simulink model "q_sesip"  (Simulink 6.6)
settings: Solver=FixedStepDiscrete  StartTime=0.0  StopTime=inf  FixedStep=0.002  RelTol=1e-3
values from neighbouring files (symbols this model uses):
  ALPHA_LIM_ENABLE = 1    [setup_srv02_exp08_sip.m]
  ALPHA_MAX = 45    [setup_srv02_exp08_sip.m]
  ALPHA_MIN = - ALPHA_MAX    (= -45)    [setup_srv02_exp08_sip.m]
  CATCH_ALPHA_DOT_LIM = VMAX_AMP/k(4)    [setup_srv02_exp08_sip.m]
  CATCH_ALPHA_UP_LIM = 1.5 * pi / 180    (= 0.0261799387799)    [setup_srv02_exp08_sip.m]
  Er = 0.8    [calculate_qr.m]
  eta_g = 0.90    (= 0.9)    [config_srv02.m]
  eta_m = 0.69    [config_srv02.m]
  g = 9.81    [config_sp.m]    (also in setup_srv02_exp08_sip.m)
  k = zeros(1,4)    [setup_srv02_exp08_sip.m]
  K_AMP = 1    [setup_srv02_exp08_sip.m]
  K_ENC = 0    [config_srv02.m]
  Kg = 0    [config_srv02.m]
  km = 0.804 / 1000 * K_RDPS2RPM    [config_srv02.m]
  kt = 1.088 * K_OZ2N * K_IN2M    [config_srv02.m]
  lp = (2 + 7/16) * K_IN2M    [config_sp.m]
  n = u_max / g    [setup_srv02_exp08_sip.m]
  Rm = 2.6    [config_srv02.m]
  THETA_LIM_ENABLE = 1    [setup_srv02_exp08_sip.m]
  THETA_MAX = 60    [setup_srv02_exp08_sip.m]
  THETA_MIN = - THETA_MAX    (= -60)    [setup_srv02_exp08_sip.m]
  VMAX_AMP = 0    [config_srv02.m]
  VMAX_DAC = 10    [setup_srv02_exp08_sip.m]
  wcf_2 = 2 * pi * 8.5    (= 53.407075111)    [setup_srv02_exp08_sip.m]
undefined symbols (not defined in the file or in its folder): HIL, Jp_cm, l_arm, m_arm, mp, qc_get_step_size
libraries: quarc_library x12, simulink_extras x6, simulink x2

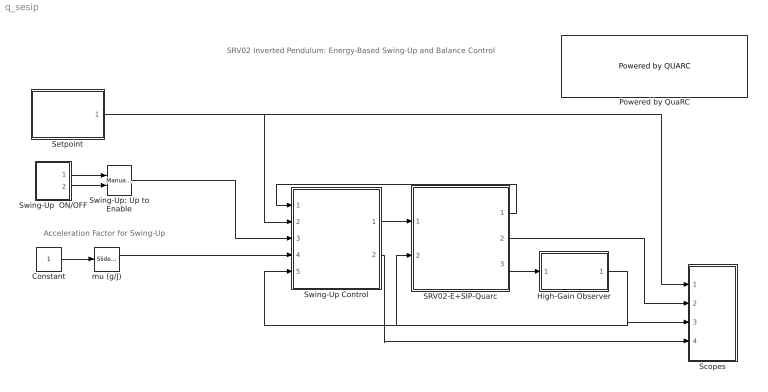
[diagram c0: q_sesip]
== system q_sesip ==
  note: SRV02 Inverted Pendulum: Energy-Based Swing-Up and Balance Control
  note: Acceleration Factor for Swing-Up
  Constant : Constant
  High-Gain Observer : Subsystem
  Powered by QuaRC : quarc_library/Logos/Powered by QUARC  SystemSampleTime=-1
  SRV02-E+SIP-Quarc : Subsystem
  Scopes : Subsystem
  Setpoint : Subsystem
  Swing-Up  ON/OFF : Subsystem
  Swing-Up Control : Subsystem
  Swing-Up: Up to Enable : simulink/Signal Routing/Manual Switch  SystemSampleTime=-1  sw=1  action=0  varsize=off
  mu (g/J) : simulink/Math Operations/Slider Gain  SystemSampleTime=-1  low=0  gain=0.23544  high=1
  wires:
  Swing-Up Control/1(tau (N.m)) -> SRV02-E+SIP-Quarc/1(tau (N.m))
  SRV02-E+SIP-Quarc/3(Y) -> High-Gain Observer/1(Y)
  Setpoint/1(Xd) -> Scopes/1(X_d), Swing-Up Control/2(Xd)
  SRV02-E+SIP-Quarc/1(a_f (rad)) -> Swing-Up Control/1(a_f (rad))
  Swing-Up  ON/OFF/1(on) -> Swing-Up: Up to Enable/1
  Swing-Up  ON/OFF/2(off) -> Swing-Up: Up to Enable/2
  Swing-Up: Up to Enable/1 -> Swing-Up Control/3(swing on/off)
  Swing-Up Control/2(E (J)) -> Scopes/4(E)
  SRV02-E+SIP-Quarc/2(Vm (V)) -> Scopes/2(Vm)
  High-Gain Observer/1(Xe) -> Swing-Up Control/5(X), SRV02-E+SIP-Quarc/2(X), Scopes/3(X)
  Constant/1 -> mu (g/J)/1
  mu (g/J)/1 -> Swing-Up Control/4(mu (g/J))

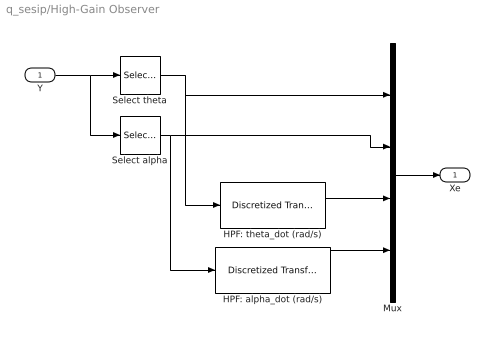
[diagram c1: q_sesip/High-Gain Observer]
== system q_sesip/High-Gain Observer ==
  Y : Inport
  HPF: alpha_dot (rad/s) : quarc_library/Discrete/Discretized Transfer Function  SystemSampleTime=-1  num=[wcf_2 0]  den=[1 wcf_2]  method=tustin  Ts=qc_get_step_size
  HPF: theta_dot (rad/s) : quarc_library/Discrete/Discretized Transfer Function  SystemSampleTime=-1  num=[100 0]  den=[1 100]  method=tustin  Ts=qc_get_step_size
  Mux : Mux
  Select alpha : Selector  IndexOptions=Index vector (dialog)  Indices=2  OutputSizes=1  InputPortWidth=2
  Select theta : Selector  IndexOptions=Index vector (dialog)  Indices=1  OutputSizes=1  InputPortWidth=2
  Xe : Outport
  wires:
  Select alpha/1 -> Mux/2, HPF: alpha_dot (rad/s)/1
  Mux/1 -> Xe/1
  Y/1 -> Select alpha/1, Select theta/1
  HPF: theta_dot (rad/s)/1 -> Mux/3
  Select theta/1 -> Mux/1, HPF: theta_dot (rad/s)/1
  HPF: alpha_dot (rad/s)/1 -> Mux/4

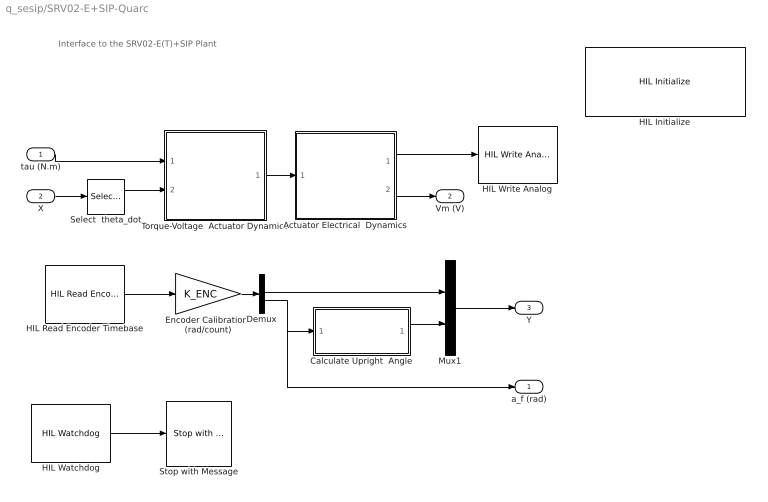
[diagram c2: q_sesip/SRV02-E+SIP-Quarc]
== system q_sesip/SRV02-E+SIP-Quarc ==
  note: Interface to the SRV02-E(T)+SIP Plant
  tau (N.m) : Inport
  X : Inport  Port=2
  Actuator Electrical  Dynamics : Subsystem
  Calculate Upright  Angle : Subsystem
  Demux : Demux  Outputs=2
  Encoder Calibration  (rad/count) : Gain  Gain=K_ENC
  HIL Initialize : quarc_library/Data Acquisition/Generic/Configuration/HIL Initialize  object_name=HIL-1  board_type=q8  board_number=0  exclusive=off  active=on  hardware_clocks=0:1  clock_modes=[0 0]  set_clock_params_at_start=on  set_clock_params_at_switch_in=off  analog_input_channels=0:7  analog_input_maximums=10  analog_input_minimums=-10  set_analog_input_params_at_start=on  set_analog_input_params_at_switch_in=off  analog_output_channels=0:7  analog_output_maximums=10  analog_output_minimums=-10  initial_analog_outputs=0  final_analog_outputs=0  watchdog_analog_outputs=0  set_analog_output_params_at_start=on  set_analog_output_params_at_switch_in=off  set_analog_outputs_at_start=on  set_analog_outputs_at_switch_in=off  set_analog_outputs_at_terminate=on  set_analog_outputs_at_switch_out=off  set_analog_outputs_on_watchdog=on  digital_input_channels=[]  digital_output_channels=[]  digital_output_configuration=[]  initial_digital_outputs=1  final_digital_outputs=1  watchdog_digital_outputs=0  set_digital_output_params_at_start=off  set_digital_output_params_at_switch_in=off  set_digital_outputs_at_start=on  set_digital_outputs_at_switch_in=off  set_digital_outputs_at_terminate=on  set_digital_outputs_at_switch_out=off  set_digital_outputs_on_watchdog=off  encoder_channels=0:7  quadrature=4  encoder_filter_frequency=(1/120e-9)/1  initial_encoder_counts=0  set_encoder_params_at_start=on  set_encoder_params_at_switch_in=off  set_encoder_counts_at_start=on  set_encoder_counts_at_switch_in=off  pwm_channels=[]  pwm_modes=0  pwm_frequency=(1/60e-9)/1024  pwm_configuration=[]  pwm_alignment=[]  pwm_polarity=[]  pwm_leading_deadband=[]  pwm_trailing_deadband=[]  initial_pwm_outputs=0  final_pwm_outputs=0  watchdog_pwm_outputs=0  set_pwm_params_at_start=on  set_pwm_params_at_switch_in=off  set_pwm_outputs_at_start=on  set_pwm_outputs_at_switch_in=off  set_pwm_outputs_at_terminate=on  set_pwm_outputs_at_switch_out=off  set_pwm_outputs_on_watchdog=off  other_output_channels=[]  initial_other_outputs=[]  final_other_outputs=[]  watchdog_other_outputs=0  set_other_outputs_at_start=on  set_other_outputs_at_switch_in=off  set_other_outputs_at_terminate=on  set_other_outputs_at_switch_out=off  set_other_outputs_on_watchdog=off
  HIL Read Encoder Timebase : quarc_library/Data Acquisition/Generic/Timebases/HIL Read Encoder Timebase  object_name=HIL-1  clock=0  channels=[0:1]  samples_in_buffer=max(ceil(1/qc_get_step_size), 1)  active=on  vector_output=on  data_type_mode=Inherit via back propagation  data_type=double
  HIL Watchdog : quarc_library/Data Acquisition/Generic/Watchdog/HIL Watchdog  object_name=HIL-1  timeout=10*qc_get_step_size  sample_time=qc_get_step_size  active=off
  HIL Write Analog : quarc_library/Data Acquisition/Generic/Immediate I//O/HIL Write Analog  object_name=HIL-1  channels=0  sample_time=-1  active=off  vector_input=off
  Mux1 : Mux  Inputs=2
  Select  theta_dot : Selector  IndexOptions=Index vector (dialog)  Indices=[3]  OutputSizes=1  InputPortWidth=4
  Stop with Message : quarc_library/Sinks/Error Handling/Stop with Message  SystemSampleTime=-1  message_type=Fixed error message  message_icon=Error  message=Stopped by watchdog.
  Torque-Voltage  Actuator Dynamics : Subsystem
  a_f (rad) : Outport
  Vm (V) : Outport  Port=2
  Y : Outport  Port=3
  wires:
  Demux/1 -> Mux1/1
  Calculate Upright  Angle/1(alpha_up) -> Mux1/2
  Mux1/1 -> Y/1
  Demux/2 -> a_f (rad)/1, Calculate Upright  Angle/1(alpha)
  Encoder Calibration  (rad/count)/1 -> Demux/1
  HIL Read Encoder Timebase/1 -> Encoder Calibration  (rad/count)/1
  tau (N.m)/1 -> Torque-Voltage  Actuator Dynamics/1(tau (N.m))
  X/1 -> Select  theta_dot/1
  Torque-Voltage  Actuator Dynamics/1(Vi (V)) -> Actuator Electrical  Dynamics/1(Vi (V))
  Select  theta_dot/1 -> Torque-Voltage  Actuator Dynamics/2(th_dot (rad/s))
  Actuator Electrical  Dynamics/2(Vm (V)) -> Vm (V)/1
  Actuator Electrical  Dynamics/1(Vdaq (V)) -> HIL Write Analog/1
  HIL Watchdog/1 -> Stop with Message/1

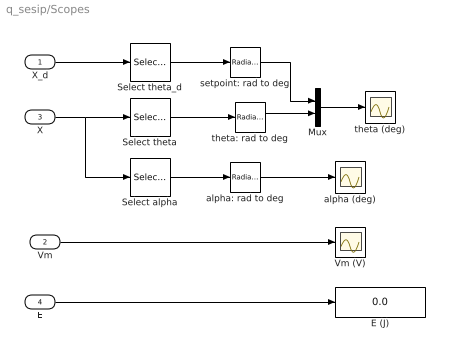
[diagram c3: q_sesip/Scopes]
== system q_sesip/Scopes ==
  X_d : Inport
  Vm : Inport  Port=2
  X : Inport  Port=3
  E : Inport  Port=4
  E (J) : Display
  Mux : Mux  Inputs=2
  Select alpha : Selector  IndexOptions=Index vector (dialog)  Indices=2  OutputSizes=1  InputPortWidth=4
  Select theta : Selector  IndexOptions=Index vector (dialog)  Indices=1  OutputSizes=1  InputPortWidth=4
  Select theta_d : Selector  IndexOptions=Index vector (dialog)  Indices=1  OutputSizes=1  InputPortWidth=4
  Vm (V) : Scope
  alpha (deg) : Scope
  alpha: rad to deg : simulink_extras/Transformations/Radians to Degrees  SystemSampleTime=-1
  setpoint: rad to deg : simulink_extras/Transformations/Radians to Degrees  SystemSampleTime=-1
  theta (deg) : Scope
  theta: rad to deg : simulink_extras/Transformations/Radians to Degrees  SystemSampleTime=-1
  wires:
  Vm/1 -> Vm (V)/1
  X_d/1 -> Select theta_d/1
  Mux/1 -> theta (deg)/1
  theta: rad to deg/1 -> Mux/2
  Select alpha/1 -> alpha: rad to deg/1
  Select theta/1 -> theta: rad to deg/1
  alpha: rad to deg/1 -> alpha (deg)/1
  X/1 -> Select alpha/1, Select theta/1
  E/1 -> E (J)/1
  setpoint: rad to deg/1 -> Mux/1
  Select theta_d/1 -> setpoint: rad to deg/1

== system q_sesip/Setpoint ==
  note: Setpoint
  Amplitude (deg) : Gain  Gain=0
  Convert to  Vector State : Gain  Gain=[1,0,0,0]
  Degrees to Radians : simulink_extras/Transformations/Degrees to Radians  SystemSampleTime=-1
  Signal Generator : SignalGenerator  WaveForm=square  Frequency=0.2
  Xd : Outport
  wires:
  Amplitude (deg)/1 -> Degrees to Radians/1
  Signal Generator/1 -> Amplitude (deg)/1
  Degrees to Radians/1 -> Convert to  Vector State/1
  Convert to  Vector State/1 -> Xd/1

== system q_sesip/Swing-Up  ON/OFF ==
  Enable Swing-Up : Constant
  No Swing-Up : Constant  Value=0
  on : Outport
  off : Outport  Port=2
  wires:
  Enable Swing-Up/1 -> on/1
  No Swing-Up/1 -> off/1

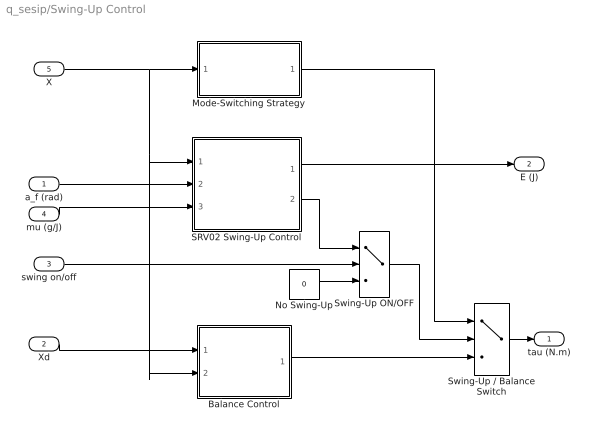
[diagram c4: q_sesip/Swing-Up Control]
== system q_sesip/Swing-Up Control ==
  a_f (rad) : Inport
  Xd : Inport  Port=2
  swing on/off : Inport  Port=3
  mu (g/J) : Inport  Port=4
  X : Inport  Port=5
  Balance Control : Subsystem
  Mode-Switching Strategy : Subsystem
  No Swing-Up : Constant  Value=0
  SRV02 Swing-Up Control : Subsystem
  Swing-Up ON/OFF : Switch  Threshold=0.5
  Swing-Up / Balance Switch : MultiPortSwitch  Inputs=2  zeroidx=on
  tau (N.m) : Outport
  E (J) : Outport  Port=2
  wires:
  Swing-Up / Balance Switch/1 -> tau (N.m)/1
  Xd/1 -> Balance Control/1(Xd)
  Swing-Up ON/OFF/1 -> Swing-Up / Balance Switch/2
  swing on/off/1 -> Swing-Up ON/OFF/2
  No Swing-Up/1 -> Swing-Up ON/OFF/3
  SRV02 Swing-Up Control/2(tau (N.m)) -> Swing-Up ON/OFF/1
  X/1 -> SRV02 Swing-Up Control/1(X), Balance Control/2(X), Mode-Switching Strategy/1(X)
  SRV02 Swing-Up Control/1(E (J)) -> E (J)/1
  a_f (rad)/1 -> SRV02 Swing-Up Control/2(a_f (rad))
  Mode-Switching Strategy/1(enable) -> Swing-Up / Balance Switch/1
  Balance Control/1(tau (N.m)) -> Swing-Up / Balance Switch/3
  mu (g/J)/1 -> SRV02 Swing-Up Control/3(mu (g/J))

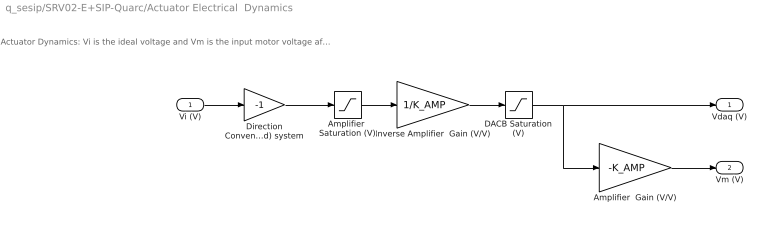
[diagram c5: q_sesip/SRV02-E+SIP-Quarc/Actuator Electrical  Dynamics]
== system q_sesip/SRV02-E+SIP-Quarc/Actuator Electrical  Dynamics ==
  note: Actuator Dynamics: Vi is the ideal voltage and Vm is the input motor voltage after going through the DACB and amplifier limitiations.
  Vi (V) : Inport
  Amplifier  Gain (V/V) : Gain  Gain=-K_AMP
  Amplifier  Saturation (V) : Saturate  UpperLimit=VMAX_AMP  LowerLimit=-VMAX_AMP
  DACB Saturation (V) : Saturate  UpperLimit=VMAX_DAC  LowerLimit=-VMAX_DAC
  Direction Convention: (Right-Hand) system : Gain  Gain=-1
  Inverse Amplifier  Gain (V/V) : Gain  Gain=1/K_AMP
  Vdaq (V) : Outport
  Vm (V) : Outport  Port=2
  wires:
  Vi (V)/1 -> Direction Convention: (Right-Hand) system/1
  Amplifier  Saturation (V)/1 -> Inverse Amplifier  Gain (V/V)/1
  Inverse Amplifier  Gain (V/V)/1 -> DACB Saturation (V)/1
  DACB Saturation (V)/1 -> Amplifier  Gain (V/V)/1, Vdaq (V)/1
  Amplifier  Gain (V/V)/1 -> Vm (V)/1
  Direction Convention: (Right-Hand) system/1 -> Amplifier  Saturation (V)/1

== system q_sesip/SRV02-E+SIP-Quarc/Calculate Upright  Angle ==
  alpha : Inport
  Math Function : Math  Operator=mod
  Mod Angle  (rad) : Constant  Value=2*pi
  Offset Angle  (rad) : Constant  Value=pi
  Sum : Sum  Inputs=+-
  alpha_up : Outport
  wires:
  Offset Angle  (rad)/1 -> Sum/2
  Math Function/1 -> Sum/1
  Mod Angle  (rad)/1 -> Math Function/2
  alpha/1 -> Math Function/1
  Sum/1 -> alpha_up/1

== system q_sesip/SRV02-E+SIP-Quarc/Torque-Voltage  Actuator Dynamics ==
  tau (N.m) : Inport
  th_dot (rad/s) : Inport  Port=2
  Back-EMF (V.s/rad) : Gain  Gain=Kg*km
  Torque to Voltage (V/(N.m)) : Gain  Gain=Rm / ( eta_g * Kg * eta_m * kt )
  Vi : Sum  OutScaling=2^-10
  Vi (V) : Outport
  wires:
  tau (N.m)/1 -> Torque to Voltage (V/(N.m))/1
  th_dot (rad/s)/1 -> Back-EMF (V.s/rad)/1
  Torque to Voltage (V/(N.m))/1 -> Vi/1
  Back-EMF (V.s/rad)/1 -> Vi/2
  Vi/1 -> Vi (V)/1

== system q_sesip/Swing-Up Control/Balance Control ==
  Xd : Inport
  X : Inport  Port=2
  PD  Control Gain : Gain  Gain=k  Multiplication=Matrix(K*u)
  Sum : Sum  Inputs=+-
  tau (N.m) : Outport
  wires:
  Sum/1 -> PD  Control Gain/1
  X/1 -> Sum/2
  Xd/1 -> Sum/1
  PD  Control Gain/1 -> tau (N.m)/1

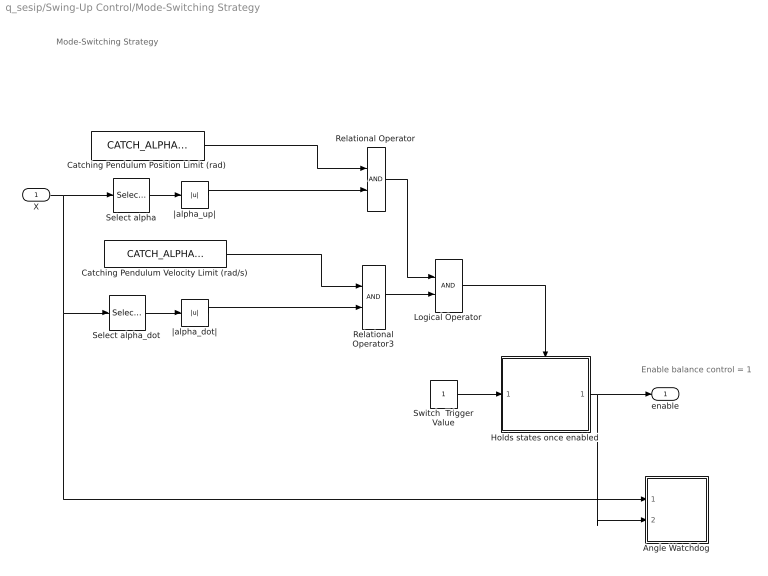
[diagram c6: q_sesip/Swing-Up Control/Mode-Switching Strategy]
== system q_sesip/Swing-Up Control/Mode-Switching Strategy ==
  note: Mode-Switching Strategy
  note: Enable balance control = 1
  X : Inport
  Angle Watchdog : Subsystem
  Catching Pendulum Position Limit (rad) : Constant  Value=CATCH_ALPHA_UP_LIM
  Catching Pendulum Velocity Limit (rad/s) : Constant  Value=CATCH_ALPHA_DOT_LIM
  Holds states once enabled : Subsystem  TreatAsAtomicUnit=on
  Logical Operator : Logic
  Relational Operator : RelationalOperator
  Relational Operator3 : RelationalOperator
  Select alpha : Selector  IndexOptions=Index vector (dialog)  Indices=2  OutputSizes=1  InputPortWidth=4
  Select alpha_dot : Selector  IndexOptions=Index vector (dialog)  Indices=4  OutputSizes=1  InputPortWidth=4
  Switch  Trigger Value : Constant
  |alpha_dot| : Abs
  |alpha_up| : Abs
  enable : Outport
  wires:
  Catching Pendulum Position Limit (rad)/1 -> Relational Operator/1
  Logical Operator/1 -> Holds states once enabled/Enable
  Relational Operator/1 -> Logical Operator/1
  Relational Operator3/1 -> Logical Operator/2
  Select alpha_dot/1 -> |alpha_dot|/1
  Catching Pendulum Velocity Limit (rad/s)/1 -> Relational Operator3/1
  |alpha_dot|/1 -> Relational Operator3/2
  Holds states once enabled/1(Sw Trigger) -> enable/1, Angle Watchdog/2(enable)
  Switch  Trigger Value/1 -> Holds states once enabled/1(Trigger)
  Select alpha/1 -> |alpha_up|/1
  |alpha_up|/1 -> Relational Operator/2
  X/1 -> Select alpha/1, Select alpha_dot/1, Angle Watchdog/1(X)

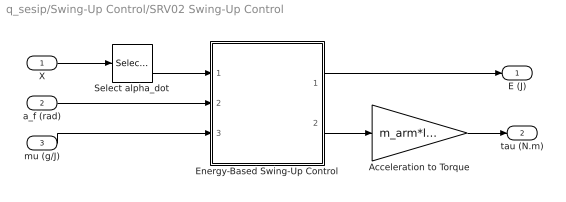
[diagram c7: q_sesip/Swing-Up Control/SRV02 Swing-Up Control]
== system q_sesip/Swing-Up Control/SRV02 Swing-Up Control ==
  X : Inport
  a_f (rad) : Inport  Port=2
  mu (g/J) : Inport  Port=3
  Acceleration to Torque : Gain  Gain=m_arm*l_arm
  Energy-Based Swing-Up Control : Subsystem
  Select alpha_dot : Selector  IndexOptions=Index vector (dialog)  Indices=4  OutputSizes=1  InputPortWidth=4
  E (J) : Outport
  tau (N.m) : Outport  Port=2
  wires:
  Energy-Based Swing-Up Control/1(E (J)) -> E (J)/1
  a_f (rad)/1 -> Energy-Based Swing-Up Control/2(a_f (rad))
  Select alpha_dot/1 -> Energy-Based Swing-Up Control/1(a_dot (rad/s))
  X/1 -> Select alpha_dot/1
  Acceleration to Torque/1 -> tau (N.m)/1
  Energy-Based Swing-Up Control/2(u (m/s^2)) -> Acceleration to Torque/1
  mu (g/J)/1 -> Energy-Based Swing-Up Control/3(mu (g/J))

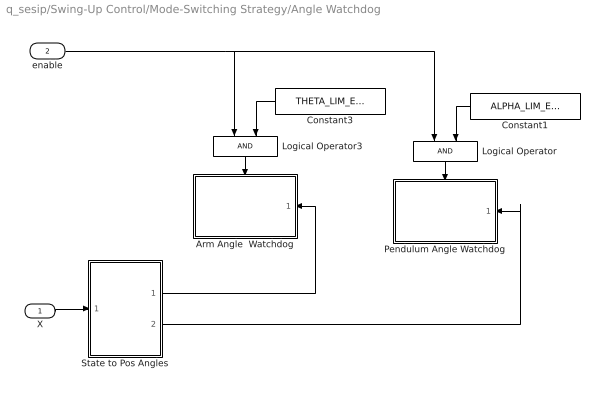
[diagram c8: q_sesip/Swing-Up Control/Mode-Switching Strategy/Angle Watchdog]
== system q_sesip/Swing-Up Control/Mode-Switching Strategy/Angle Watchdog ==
  X : Inport
  enable : Inport  Port=2
  Arm Angle  Watchdog : Subsystem  Orientation=left  TreatAsAtomicUnit=on
  Constant1 : Constant  Orientation=left  Value=ALPHA_LIM_ENABLE
  Constant3 : Constant  Orientation=left  Value=THETA_LIM_ENABLE
  Logical Operator : Logic  Orientation=down
  Logical Operator3 : Logic  Orientation=down
  Pendulum Angle Watchdog : Subsystem  Orientation=left  TreatAsAtomicUnit=on
  State to Pos Angles : Subsystem
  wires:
  State to Pos Angles/2(alpha (rad)) -> Pendulum Angle Watchdog/1(alpha (rad))
  State to Pos Angles/1(theta (rad)) -> Arm Angle  Watchdog/1(theta (rad))
  enable/1 -> Logical Operator/1, Logical Operator3/1
  X/1 -> State to Pos Angles/1(X)
  Logical Operator/1 -> Pendulum Angle Watchdog/Enable
  Constant1/1 -> Logical Operator/2
  Logical Operator3/1 -> Arm Angle  Watchdog/Enable
  Constant3/1 -> Logical Operator3/2

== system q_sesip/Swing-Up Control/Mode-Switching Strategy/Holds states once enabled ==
  Trigger : Inport
  Enable : EnablePort
  Sw Trigger : Outport  InitialOutput=[0]
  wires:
  Trigger/1 -> Sw Trigger/1

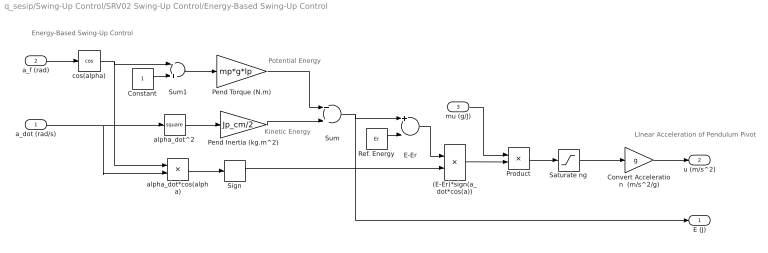
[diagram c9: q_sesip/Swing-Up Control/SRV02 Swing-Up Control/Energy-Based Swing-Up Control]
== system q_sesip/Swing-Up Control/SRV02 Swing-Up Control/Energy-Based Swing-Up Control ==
  note: Energy-Based Swing-Up Control
  note: Kinetic Energy
  note: Potential Energy
  note: LInear Acceleration of Pendulum Pivot
  a_dot (rad/s) : Inport
  a_f (rad) : Inport  Port=2
  mu (g/J) : Inport  Port=3
  (E-Er)*sign(a_dot*cos(a)) : Product
  Constant : Constant
  Convert Acceleration  (m/s^2/g) : Gain  Gain=g
  E-Er : Sum  Inputs=+-  OutScaling=2^-10
  Pend Inertia (kg.m^2) : Gain  Gain=Jp_cm/2
  Pend Torque (N.m) : Gain  Gain=mp*g*lp
  Product : Product
  Ref. Energy : Constant  Value=Er
  Saturate ng : Saturate  UpperLimit=n*g  LowerLimit=-n*g
  Sign : Signum
  Sum : Sum
  Sum1 : Sum  Inputs=-+
  alpha_dot*cos(alpha) : Product
  alpha_dot^2 : Math  Operator=square
  cos(alpha) : Trigonometry  Operator=cos
  E (J) : Outport
  u (m/s^2) : Outport  Port=2
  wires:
  alpha_dot*cos(alpha)/1 -> Sign/1
  Sign/1 -> (E-Er)*sign(a_dot*cos(a))/2
  Saturate ng/1 -> Convert Acceleration  (m/s^2/g)/1
  Constant/1 -> Sum1/2
  cos(alpha)/1 -> alpha_dot*cos(alpha)/1, Sum1/1
  a_f (rad)/1 -> cos(alpha)/1
  E-Er/1 -> (E-Er)*sign(a_dot*cos(a))/1
  Sum/1 -> E (J)/1, E-Er/1
  Pend Inertia (kg.m^2)/1 -> Sum/2
  Sum1/1 -> Pend Torque (N.m)/1
  alpha_dot^2/1 -> Pend Inertia (kg.m^2)/1
  Pend Torque (N.m)/1 -> Sum/1
  a_dot (rad/s)/1 -> alpha_dot^2/1, alpha_dot*cos(alpha)/2
  Convert Acceleration  (m/s^2/g)/1 -> u (m/s^2)/1
  (E-Er)*sign(a_dot*cos(a))/1 -> Product/2
  Product/1 -> Saturate ng/1
  Ref. Energy/1 -> E-Er/2
  mu (g/J)/1 -> Product/1

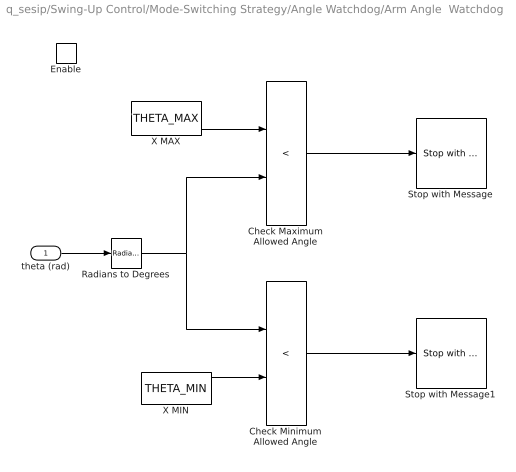
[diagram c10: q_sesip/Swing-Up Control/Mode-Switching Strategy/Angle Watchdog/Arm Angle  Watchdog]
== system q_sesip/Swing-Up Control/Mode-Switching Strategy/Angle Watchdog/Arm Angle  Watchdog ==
  theta (rad) : Inport
  Enable : EnablePort
  Check Maximum Allowed Angle : RelationalOperator  Operator=<
  Check Minimum Allowed Angle : RelationalOperator  Operator=<
  Radians to Degrees : simulink_extras/Transformations/Radians to Degrees  SystemSampleTime=-1
  Stop with Message : quarc_library/Sinks/Error Handling/Stop with Message  SystemSampleTime=-1  message_type=Fixed error message  message_icon=Error  message=Maximum arm angle reached.
  Stop with Message1 : quarc_library/Sinks/Error Handling/Stop with Message  SystemSampleTime=-1  message_type=Fixed error message  message_icon=Error  message=Minimum arm angle reached.
  X MAX : Constant  Value=THETA_MAX
  X MIN : Constant  Value=THETA_MIN
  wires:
  Radians to Degrees/1 -> Check Minimum Allowed Angle/1, Check Maximum Allowed Angle/2
  theta (rad)/1 -> Radians to Degrees/1
  X MIN/1 -> Check Minimum Allowed Angle/2
  X MAX/1 -> Check Maximum Allowed Angle/1
  Check Maximum Allowed Angle/1 -> Stop with Message/1
  Check Minimum Allowed Angle/1 -> Stop with Message1/1

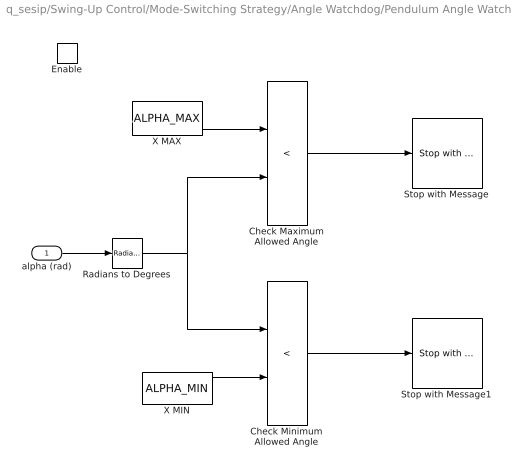
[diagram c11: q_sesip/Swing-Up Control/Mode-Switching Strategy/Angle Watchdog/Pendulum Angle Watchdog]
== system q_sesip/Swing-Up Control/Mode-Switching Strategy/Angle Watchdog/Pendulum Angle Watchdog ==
  alpha (rad) : Inport
  Enable : EnablePort
  Check Maximum Allowed Angle : RelationalOperator  Operator=<
  Check Minimum Allowed Angle : RelationalOperator  Operator=<
  Radians to Degrees : simulink_extras/Transformations/Radians to Degrees  SystemSampleTime=-1
  Stop with Message : quarc_library/Sinks/Error Handling/Stop with Message  SystemSampleTime=-1  message_type=Fixed error message  message_icon=Error  message=Maximum pendulum angle reached.
  Stop with Message1 : quarc_library/Sinks/Error Handling/Stop with Message  SystemSampleTime=-1  message_type=Fixed error message  message_icon=Error  message=Minimum pendulum angle reached.
  X MAX : Constant  Value=ALPHA_MAX
  X MIN : Constant  Value=ALPHA_MIN
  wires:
  X MAX/1 -> Check Maximum Allowed Angle/1
  X MIN/1 -> Check Minimum Allowed Angle/2
  alpha (rad)/1 -> Radians to Degrees/1
  Radians to Degrees/1 -> Check Maximum Allowed Angle/2, Check Minimum Allowed Angle/1
  Check Maximum Allowed Angle/1 -> Stop with Message/1
  Check Minimum Allowed Angle/1 -> Stop with Message1/1

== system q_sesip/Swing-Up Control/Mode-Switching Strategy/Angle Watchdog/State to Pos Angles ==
  X : Inport
  Select alpha : Selector  IndexOptions=Index vector (dialog)  Indices=2  OutputSizes=1  InputPortWidth=4
  Select theta : Selector  IndexOptions=Index vector (dialog)  Indices=1  OutputSizes=1  InputPortWidth=4
  |alpha| : Abs
  |theta| : Abs
  theta (rad) : Outport
  alpha (rad) : Outport  Port=2
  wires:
  Select alpha/1 -> |alpha|/1
  Select theta/1 -> |theta|/1
  X/1 -> Select alpha/1, Select theta/1
  |theta|/1 -> theta (rad)/1
  |alpha|/1 -> alpha (rad)/1
